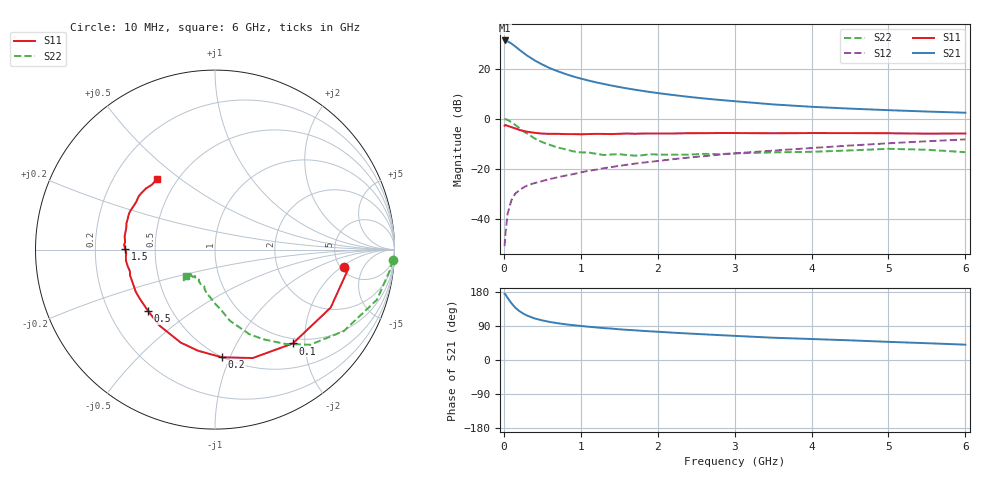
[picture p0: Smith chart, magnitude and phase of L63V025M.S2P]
!  INFINEON TECHNOLOGIES Small Signal Semiconductors
! BFR380L3 , Si-NPN RF-Transistor in TSLP-3-1
!  Vce=3 V,  Ic=25 mA
! Common Emitter S-Parameters:  07. March 2005
#  GHz  S  MA  R  50
! f  S11  S21  S12  S22
! GHz  Mag  Ang  Mag  Ang  Mag  Ang  Mag  Ang
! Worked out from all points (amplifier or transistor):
!   36 points, 10 MHz to 6 GHz, reference 50 ohm
!   highest |S21| = 31.2 dB at 10 MHz (marker M1)
!   |S21| within 3 dB of that: start of sweep to 173.4 MHz
!   unconditionally stable (mu >= 1): 1.852 GHz to 4.784 GHz
!   at 250 MHz: K = 0.40, MSG = 26.9 dB, |S12| = -27.5 dB
!   at 1.4 GHz: K = 0.96, MSG = 16.2 dB, |S12| = -19.2 dB
!   at 6 GHz: K = 0.98, MSG = 5.3 dB, |S12| = -8.2 dB
!   S11 on the Smith chart (normalised r, x): 10 MHz: 5.37, -2.25; 100 MHz: 0.91, -1.76; 200 MHz: 0.50, -0.93; 500 MHz: 0.37, -0.34; 1.5 GHz: 0.33, +0.01; 6 GHz: 0.39, +0.41
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0.01  0.7275 -7.8  36.19 174.7  0.0029 81.0  0.9932 -3.4
0.02  0.7508 -8.1  35.85 173.4  0.005 89.1  0.9793 -7.1
0.05  0.7211 -26.6  34.67 163.5  0.013 79.3  0.9445 -17.2
0.1  0.6794 -50.3  31.23 149.5  0.0243 68.1  0.8494 -32.3
0.15  0.6397 -70.8  27.39 137.9  0.0325 61.4  0.75 -45.0
0.2  0.6011 -86.4  23.75 129.3  0.0375 58.6  0.6542 -53.4
0.25  0.5716 -99.4  20.75 122.8  0.0422 55.0  0.5664 -61.8
0.3  0.5523 -110.2  18.18 117.4  0.0466 53.2  0.5084 -67.9
0.4  0.5242 -126.3  14.54 109.7  0.0524 51.7  0.4055 -78.1
0.5  0.5057 -137.4  12.01 104.5  0.0574 53.0  0.3409 -83.9
0.6  0.5005 -146.1  10.14 100.3  0.063 54.3  0.3009 -89.9
0.8  0.4946 -158.0  7.789 94.2  0.0737 56.9  0.2463 -101.2
0.9  0.4948 -163.1  6.949 91.9  0.0788 58.0  0.2245 -105.2
1.1  0.4954 -169.5  5.759 87.8  0.0918 60.2  0.2126 -111.0
1.5  0.5015 179.3  4.281 81.0  0.1154 62.5  0.1964 -121.3
1.8  0.5063 173.1  3.591 76.9  0.133 63.3  0.1874 -126.6
2.2  0.5086 166.5  2.967 72.1  0.1566 64.0  0.1924 -130.0
2.8  0.5196 157.4  2.372 65.7  0.192 64.3  0.1973 -136.6
3.5  0.5129 148.7  1.929 58.8  0.2316 62.8  0.2141 -136.0
4.5  0.517 142.4  1.59 51.9  0.2926 61.6  0.2338 -135.7
5.5  0.5044 134.3  1.391 44.3  0.3556 58.1  0.2413 -135.6
6  0.5085 129.2  1.317 40.5  0.3882 56.1  0.2157 -137.5
